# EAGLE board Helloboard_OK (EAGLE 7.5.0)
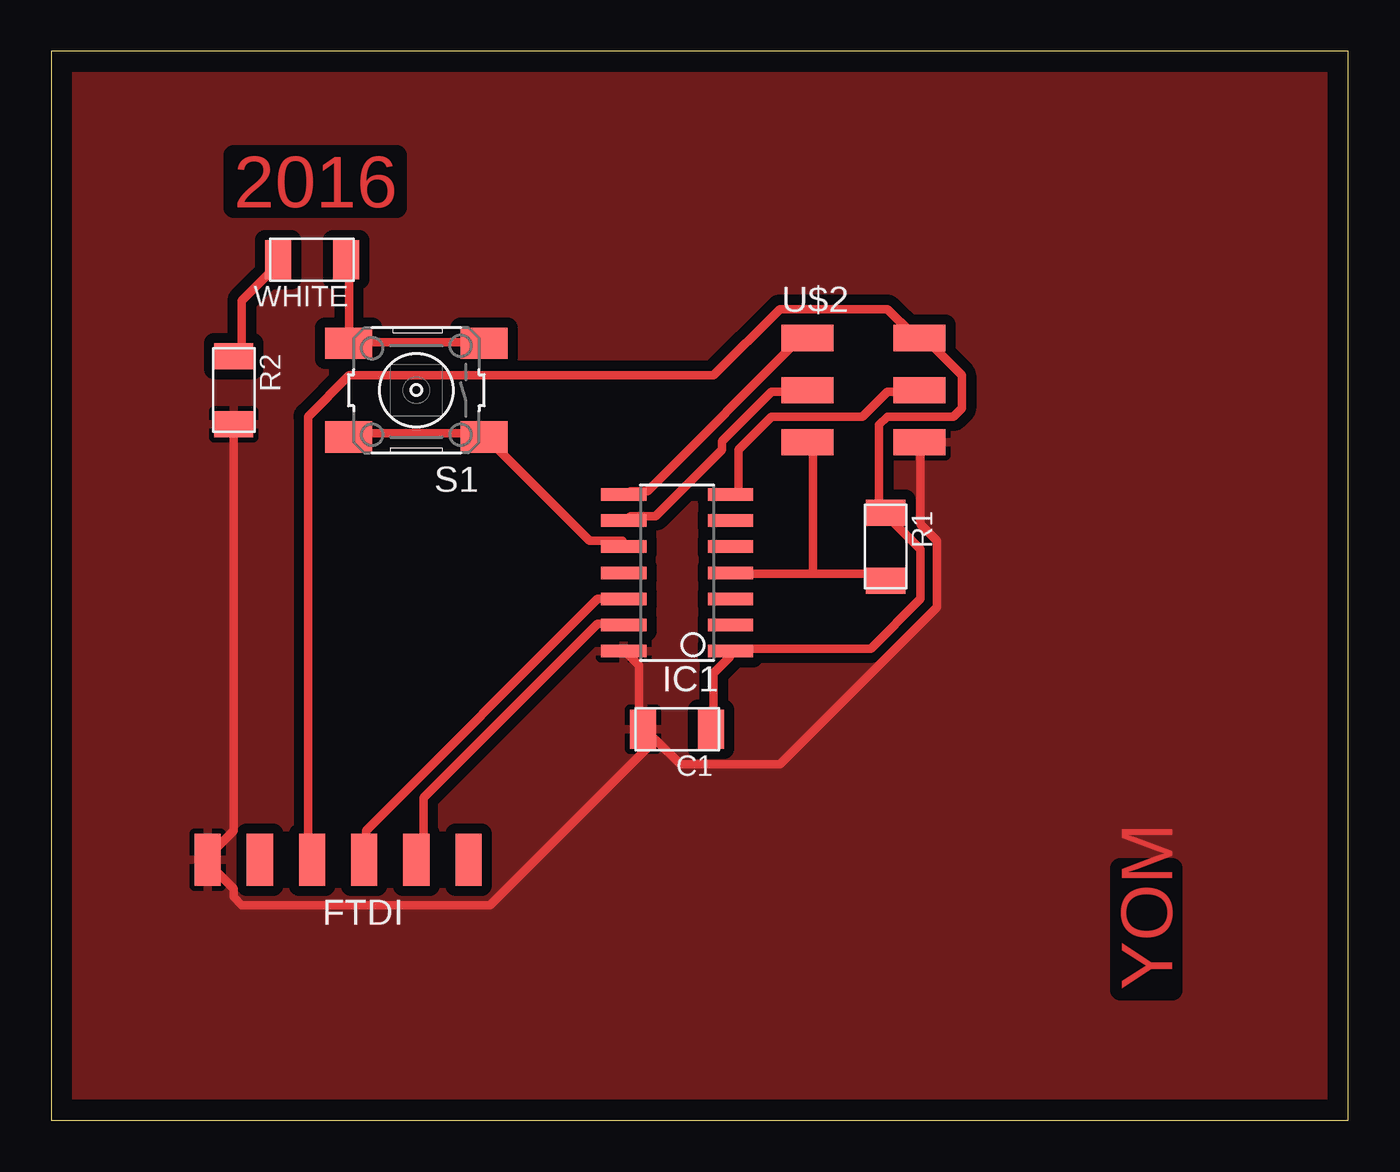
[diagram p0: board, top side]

Size 63.17 x 52.06 mm. Coordinates in mm from the lower left corner, seen from the top.
Outline: 0,0 63.17,0 63.17,52.06 0,52.06 0,0
Copper layers (1*16): Top 0.035mm / dielectric 1.5mm / Bottom 0.035mm
Design rules "default *": minimum track width 16mil, minimum drill 24mil, track to track 0.4mm, track to pad 0.4mm, pad to pad 0.4mm, via to via 0.4mm, smd to smd 8mil, copper to edge 40mil, drill to drill 8mil, minimum pad ring 10mil, minimum via ring 8mil, stop-mask expansion 4mil, vias tented up to drill 0mil, thermal gap 10mil

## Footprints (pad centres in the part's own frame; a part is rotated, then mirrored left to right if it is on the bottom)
C1206FAB = smd 1.27 x 1.905: 1 -1.651,0; 2 1.651,0
1X06SMD = smd 2.54 x 1.27: 1 0,6.35; 2 0,3.81; 3 0,1.27; 4 0,-1.27; 5 0,-3.81; 6 0,-6.35
SOIC14 = smd 0.61 x 2.21: 1 -3.81,-2.603; 2 -2.54,-2.603; 3 -1.27,-2.603; 4 0,-2.603; 5 1.27,-2.603; 6 2.54,-2.603; 7 3.81,-2.603; 8 3.81,2.603; 9 2.54,2.603; 10 1.27,2.603; 11 0,2.603; 12 -1.27,2.603; 13 -2.54,2.603; 14 -3.81,2.603
R1206FAB = smd 1.27 x 1.905: 1 -1.651,0; 2 1.651,0
6MM_SWITCH = smd 2.286 x 1.524: 1 -3.302,2.286; 2 3.302,2.286; 3 -3.302,-2.286; 4 3.302,-2.286
2X03SMD = smd 2.54 x 1.27: 1 -2.54,2.54; 2 2.92,2.54; 3 -2.54,0; 4 2.92,0; 5 -2.54,-2.54; 6 2.92,-2.54
LED1206FAB = smd 1.27 x 1.905: 1 -1.651,0; 2 1.651,0

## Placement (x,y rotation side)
C1  1uF  [C1206FAB]  30.48,19.05 180 top
FTDI  FTDI-SMD-HEADER  [1X06SMD]  13.97,12.7 90 top
IC1  ATTINY44-SSU  [SOIC14]  30.48,26.67 90 top
R1  10k  [R1206FAB]  40.64,27.94 270 top
R2  50ohm  [R1206FAB]  8.89,35.56 270 top
S1  5V  [6MM_SWITCH]  17.78,35.56 180 top
U$2  AVRISPSMD  [2X03SMD]  39.37,35.56 0 top
WHITE  LEDFAB1206  [LED1206FAB]  12.7,41.91 180 top

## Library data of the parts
C1 FTDI IC1 R1 S1 U$2 WHITE = fab
R2 = fab; R2: 50OHM

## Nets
GND: C1.2 FTDI.1 IC1.14 R2.2 U$2.6
LED: IC1.10 S1.1 S1.2
MISO: IC1.8 U$2.1
MOSI: IC1.7 U$2.4
N$1: R2.1 WHITE.2
N$2: S1.3 S1.4 WHITE.1
RST: IC1.4 R1.2 U$2.5
RX: FTDI.5 IC1.13
SCK: IC1.9 U$2.3
TX: FTDI.4 IC1.12
VCC: C1.1 FTDI.3 IC1.1 R1.1 U$2.2
XTAL1: IC1.2
XTAL2: IC1.3

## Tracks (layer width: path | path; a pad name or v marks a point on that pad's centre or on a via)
GND
  Top 0.406: R2.2 8.87,33.87 8.87,14.11 7.66,12.9 FTDI.1 7.66,12.5 8.87,11.29 8.87,10.89 9.27,10.48 21.37,10.48 29.43,18.55 | C1.2 28.63,19.35 28.63,22.18 28.22,22.58 IC1.14 | 29.43,18.55 29.03,18.95 C1.2 | 29.43,18.55 30.64,17.34 35.48,17.34 43.14,25 43.14,28.22 42.34,29.03 42.34,32.66 U$2.6 | 29.43,18.55 C1.2
  pour Top (isolate 0.5): -3.81,54.61 67.31,54.61 67.31,-3.81 -3.81,-3.81
LED
  Top 0.406: IC1.10 27.82,28.22 26.21,28.22 21.37,33.06 S1.1 20.97,33.47 14.52,33.47 S1.2
MISO
  Top 0.406: IC1.8 28.22,30.64 29.03,30.64 36.69,38.3 U$2.1
MOSI
  Top 0.406: IC1.7 33.47,30.64 33.47,32.66 35.08,34.27 39.51,34.27 40.72,35.48 41.93,35.48 U$2.4
N$1
  Top 0.406: R2.1 9.27,37.5 9.27,39.92 10.89,41.53 WHITE.2
N$2
  Top 0.406: 14.52,37.9 14.52,41.53 WHITE.1 | 14.52,37.9 20.97,37.9 S1.3 | 14.52,37.9 S1.4
RST
  Top 0.406: 37.09,26.61 33.47,26.61 IC1.4 | 37.09,26.61 40.32,26.61 R1.2 | 37.09,26.61 37.09,32.66 U$2.5
RX
  Top 0.406: IC1.13 27.82,24.19 26.61,24.19 18.14,15.72 18.14,12.9 FTDI.5
SCK
  Top 0.406: IC1.9 28.22,29.43 29.43,29.43 32.66,32.66 32.66,33.06 35.08,35.48 36.69,35.48 U$2.3
TX
  Top 0.406: IC1.12 27.82,25.4 26.61,25.4 15.32,14.11 15.32,12.9 FTDI.4
VCC
  Top 0.406: C1.1 32.26,19.35 32.26,21.77 33.06,22.58 IC1.1 33.47,22.98 39.92,22.98 42.34,25.4 42.34,27.82 40.72,29.43 R1.1 40.32,29.84 40.32,33.87 40.72,34.27 43.95,34.27 44.35,34.67 44.35,36.29 42.34,38.3 U$2.2 41.93,38.3 40.72,39.51 35.48,39.51 32.26,36.29 14.52,36.29 12.5,34.27 12.5,12.9 FTDI.3

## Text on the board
Top: 2016 | YOM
